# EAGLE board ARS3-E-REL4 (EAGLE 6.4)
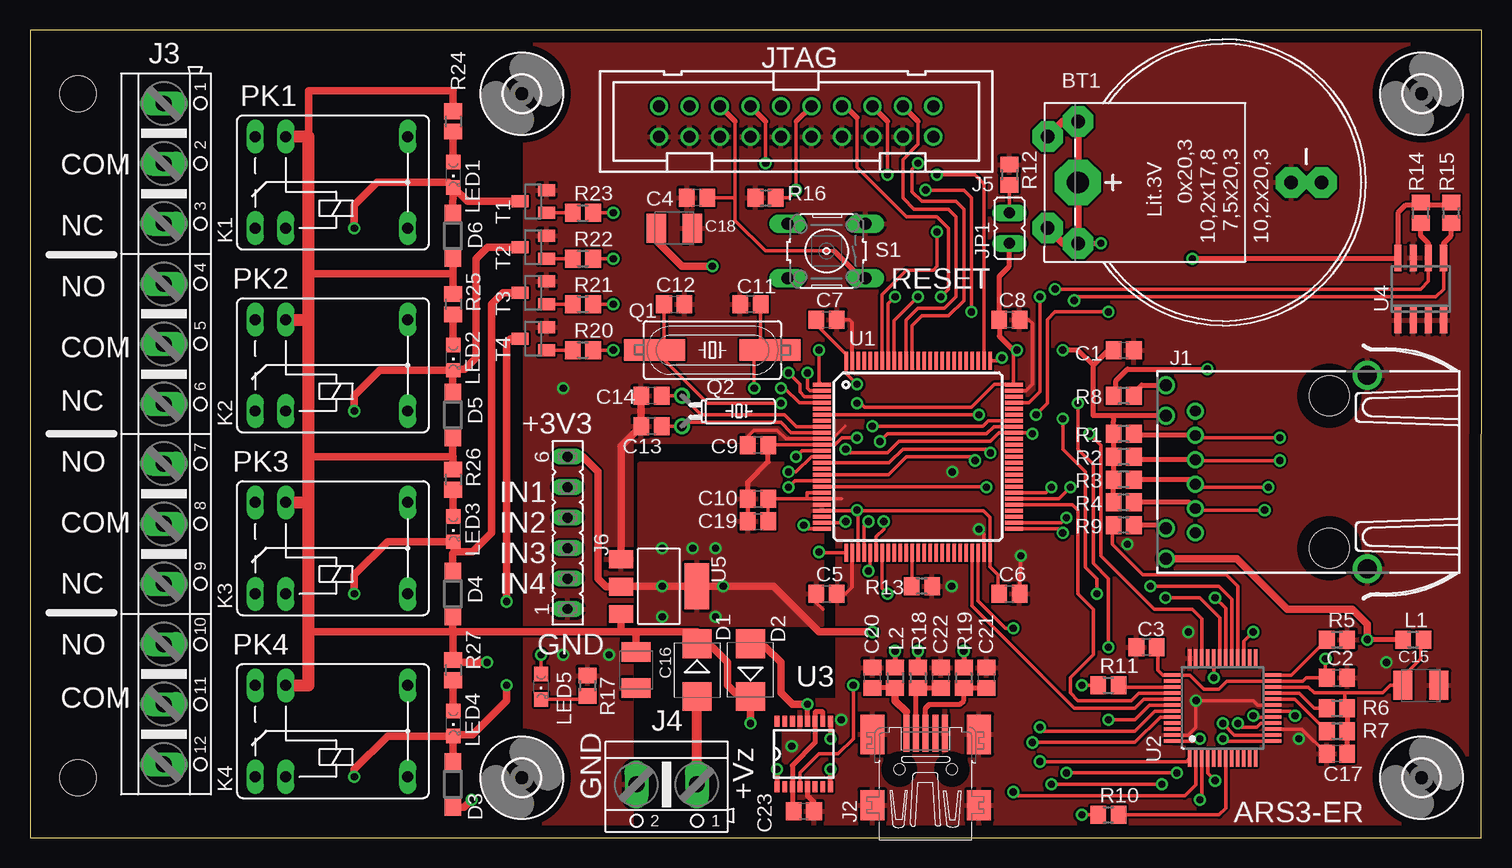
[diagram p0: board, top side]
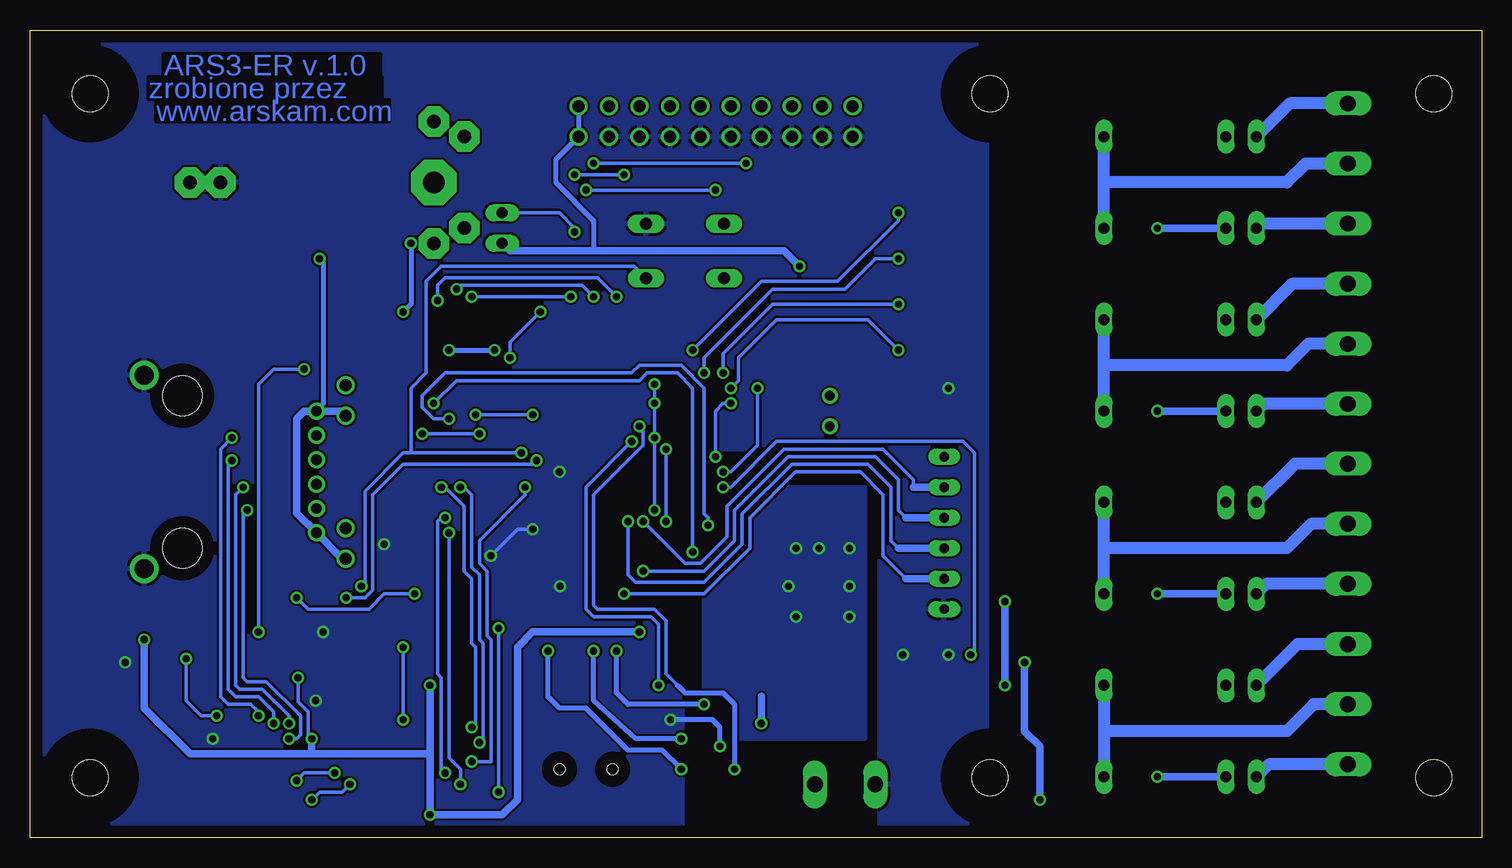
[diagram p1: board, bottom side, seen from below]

Size 121.02 x 67.31 mm. Coordinates in mm from the lower left corner, seen from the top.
Outline: 0,0 121,0 121.02,67.31 0,67.31 0,0
Copper layers (1*16): Top 0.035mm / dielectric 1.5mm / Bottom 0.035mm
Design rules "default *": minimum track width 10mil, minimum drill 19mil, track to track 7mil, track to pad 7mil, pad to pad 7mil, via to via 7mil, smd to smd 7mil, copper to edge 40mil, drill to drill 8mil, minimum pad ring 10mil, minimum via ring 8mil, stop-mask expansion 4mil, vias tented up to drill 0mil, thermal gap 10mil
Holes 3 mm at 4,5 4,62

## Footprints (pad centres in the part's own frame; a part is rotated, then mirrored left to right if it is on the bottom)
B2430UNI = drill 1.118 pad 2.54 octagon: + 3.81,14.605; +@1 -3.81,14.605; +@2 -5.08,12.065; +@3 5.08,12.065; - 0,-5.715; -@1 0,-8.255 | drill 1.803 pad 3.81 octagon: +@4 0,12.065
C0805 = smd 1.3 x 1.5: 1 -0.85,0; 2 0.85,0
SMC_B = smd 1.6 x 2.4: + -1.5,0; - 1.5,0
SMB = smd 2.4 x 2.4: A 2.2,0; C -2.2,0
SOD123 = smd 1.4 x 1.4: A 1.9,0; C -1.9,0
JP = drill 0.9 pad 1.3: 1 5.075,11.18; 2 3.045,11.18; 3 1.015,11.18; 4 -1.015,11.18; 5 -3.045,11.18; 6 -5.075,11.18 | drill 1 pad 1.4: 7 7.23,13.62; 8 4.69,13.62; 9 -4.69,13.62; 10 -7.23,13.62 | drill 1.6 pad 2.184: SH1 -8.065,-3.17; SH2 8.065,-3.17 | hole 3.3: 6.35,0; -6.35,0
32005-201 = smd 3.1 x 0.5: 1 3,1.6; 2 3,0.8; 3 3,0; 4 3,-0.8; 5 3,-1.6 | smd 2.5 x 2: M1 -3,-4.45; M2 -3,4.45 | smd 3.3 x 2: M3 2.9,4.45; M4 2.9,-4.45 | hole 0.9: 0,2.2; 0,-2.2
AK500/12 = drill 1.321 long: 1 -27.534,0; 2 -22.53,0; 3 -17.526,0; 4 -12.497,0; 5 -7.493,0; 6 -2.489,0; 7 2.489,0; 8 7.493,0; 9 12.497,0; 10 17.526,0; 11 22.53,0; 12 27.534,0
AK500/2 = drill 1.321 long: 1 -2.515,0; 2 2.515,0
PAK100/2500-20 = drill 1 pad 1.422: 1 -11.43,-1.27; 2 -11.43,1.27; 3 -8.89,-1.27; 4 -8.89,1.27; 5 -6.35,-1.27; 6 -6.35,1.27; 7 -3.81,-1.27; 8 -3.81,1.27; 9 -1.27,-1.27; 10 -1.27,1.27; 11 1.27,-1.27; 12 1.27,1.27; 13 3.81,-1.27; 14 3.81,1.27; 15 6.35,-1.27; 16 6.35,1.27; 17 8.89,-1.27; 18 8.89,1.27; 19 11.43,-1.27; 20 11.43,1.27
FE06 = drill 0.813 long: 1 -6.35,0; 2 -3.81,0; 3 -1.27,0; 4 1.27,0; 5 3.81,0; 6 6.35,0
JP1 = drill 0.914 long: 1 0,-1.27; 2 0,1.27
FRS1B = drill 0.914 long: 1 0,3.81; 2 0,-3.81; O -2.54,-3.81; P 10.16,3.81; P@ 10.16,-3.81; S -2.54,3.81
R0805 = smd 1.3 x 1.5: 1 -0.85,0; 2 0.85,0
CHIPLED_0805 = smd 1.2 x 1.2: A 0,-1.05; C 0,1.05
SM49 = smd 5.08 x 1.778: 1 -4.826,0; 2 4.826,0
TC26H = drill 0.813: 1 -1.27,0; 2 1.27,0
B3F-10XX = drill 1.016 long: 1 -3.251,2.261; 2 3.251,2.261; 3 -3.251,-2.261; 4 3.251,-2.261
SOT23 = smd 1 x 1.4: 1 -0.95,-1.1; 2 0.95,-1.1; 3 0,1.1
TQFP100 = smd 1.5 x 0.3: 1 -8,6; 2 -8,5.5; 3 -8,5; 4 -8,4.5; 5 -8,4; 6 -8,3.5; 7 -8,3; 8 -8,2.5; 9 -8,2; 10 -8,1.5; 11 -8,1; 12 -8,0.5; 13 -8,0; 14 -8,-0.5; 15 -8,-1; 16 -8,-1.5; 17 -8,-2; 18 -8,-2.5; 19 -8,-3; 20 -8,-3.5; 21 -8,-4; 22 -8,-4.5; 23 -8,-5; 24 -8,-5.5; 25 -8,-6; 51 8,-6; 52 8,-5.5; 53 8,-5; 54 8,-4.5; 55 8,-4; 56 8,-3.5; 57 8,-3; 58 8,-2.5; 59 8,-2; 60 8,-1.5; 61 8,-1; 62 8,-0.5; 63 8,0; 64 8,0.5; 65 8,1; 66 8,1.5; 67 8,2; 68 8,2.5; 69 8,3; 70 8,3.5; 71 8,4; 72 8,4.5; 73 8,5; 74 8,5.5; 75 8,6 | smd 0.3 x 1.5: 26 -6,-8; 27 -5.5,-8; 28 -5,-8; 29 -4.5,-8; 30 -4,-8; 31 -3.5,-8; 32 -3,-8; 33 -2.5,-8; 34 -2,-8; 35 -1.5,-8; 36 -1,-8; 37 -0.5,-8; 38 0,-8; 39 0.5,-8; 40 1,-8; 41 1.5,-8; 42 2,-8; 43 2.5,-8; 44 3,-8; 45 3.5,-8; 46 4,-8; 47 4.5,-8; 48 5,-8; 49 5.5,-8; 50 6,-8; 76 6,8; 77 5.5,8; 78 5,8; 79 4.5,8; 80 4,8; 81 3.5,8; 82 3,8; 83 2.5,8; 84 2,8; 85 1.5,8; 86 1,8; 87 0.5,8; 88 0,8; 89 -0.5,8; 90 -1,8; 91 -1.5,8; 92 -2,8; 93 -2.5,8; 94 -3,8; 95 -3.5,8; 96 -4,8; 97 -4.5,8; 98 -5,8; 99 -5.5,8; 100 -6,8
LQFP48 = smd 1.5 x 0.3: 1 -4.15,2.75; 2 -4.15,2.25; 3 -4.15,1.75; 4 -4.15,1.25; 5 -4.15,0.75; 6 -4.15,0.25; 7 -4.15,-0.25; 8 -4.15,-0.75; 9 -4.15,-1.25; 10 -4.15,-1.75; 11 -4.15,-2.25; 12 -4.15,-2.75; 25 4.15,-2.75; 26 4.15,-2.25; 27 4.15,-1.75; 28 4.15,-1.25; 29 4.15,-0.75; 30 4.15,-0.25; 31 4.15,0.25; 32 4.15,0.75; 33 4.15,1.25; 34 4.15,1.75; 35 4.15,2.25; 36 4.15,2.75 | smd 0.3 x 1.5: 13 -2.75,-4.15; 14 -2.25,-4.15; 15 -1.75,-4.15; 16 -1.25,-4.15; 17 -0.75,-4.15; 18 -0.25,-4.15; 19 0.25,-4.15; 20 0.75,-4.15; 21 1.25,-4.15; 22 1.75,-4.15; 23 2.25,-4.15; 24 2.75,-4.15; 37 2.75,4.15; 38 2.25,4.15; 39 1.75,4.15; 40 1.25,4.15; 41 0.75,4.15; 42 0.25,4.15; 43 -0.25,4.15; 44 -0.75,4.15; 45 -1.25,4.15; 46 -1.75,4.15; 47 -2.25,4.15; 48 -2.75,4.15
SSOP16 = smd 0.914 x 0.406: 1 -2.718,2.223; 2 -2.718,1.587; 3 -2.718,0.953; 4 -2.718,0.318; 5 -2.718,-0.318; 6 -2.718,-0.953; 7 -2.718,-1.587; 8 -2.718,-2.223; 9 2.718,-2.223; 10 2.718,-1.587; 11 2.718,-0.953; 12 2.718,-0.318; 13 2.718,0.318; 14 2.718,0.953; 15 2.718,1.587; 16 2.718,2.223
SO-08 = smd 0.6 x 2.2: 1 -1.905,-2.6; 2 -0.635,-2.6; 3 0.635,-2.6; 4 1.905,-2.6; 5 1.905,2.6; 6 0.635,2.6; 7 -0.635,2.6; 8 -1.905,2.6
SOT223 = smd 1.499 x 2.007: 1 -2.261,-3.15; 2 0.025,-3.15; 3 2.311,-3.15 | smd 3.81 x 2.007: 4 0,3.15
3,0 = hole 3: 0,0

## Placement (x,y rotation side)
BT1  [B2430UNI]  99.42,54.61 90 top
C1  100n  [C0805]  91.17,40.64 0 top
C2  100n  [C0805]  108.95,13.34 0 top
C3  100n  [C0805]  93.08,15.88 180 top
C4  100n  [C0805]  55.61,53.34 180 top
C5  100n  [C0805]  66.41,20.32 0 top
C6  100n  [C0805]  81.64,20.32 0 top
C7  100n  [C0805]  66.41,43.18 0 top
C8  100n  [C0805]  81.64,43.18 0 top
C9  100n  [C0805]  60.69,32.7 180 top
C10  100n  [C0805]  60.69,28.26 0 top
C11  15p  [C0805]  60.05,44.45 180 top
C12  15p  [C0805]  53.7,44.45 0 top
C13  15p  [C0805]  51.8,34.29 180 top
C14  15p  [C0805]  51.8,36.83 180 top
C15  10u/16  [SMC_B]  115.94,12.7 0 top
C16  10u/16  [SMC_B]  50.53,13.97 270 top
C17  100n  [C0805]  108.95,6.99 180 top
C18  10u/16  [SMC_B]  53.7,50.8 0 top
C19  100n  [C0805]  60.69,26.35 0 top
C20  10n  [C0805]  70.22,13.34 90 top
C21  47p  [C0805]  79.74,13.34 90 top
C22  47p  [C0805]  75.93,13.34 90 top
C23  100n  [C0805]  64.5,2.22 0 top
D1  [SMB]  55.61,13.97 270 top
D2  [SMB]  60.05,13.97 90 top
D3  MBR0530T1G  [SOD123]  35.24,4.45 90 top
D4  MBR0530T1G  [SOD123]  35.24,20.32 90 top
D5  MBR0530T1G  [SOD123]  35.24,35.24 90 top
D6  MBR0530T1G  [SOD123]  35.24,50.16 90 top
J1  [JP]  108.31,30.48 90 top
J2  MINI-USB  [32005-201]  74.66,5.71 90 top
J3  [AK500/12]  11.16,33.66 270 top
J4  DG301-5.0/2  [AK500/2]  53.07,4.45 180 top
J5  [PAK100/2500-20]  63.87,59.69 180 top
J6  [FE06]  44.81,25.4 90 top
JP1  ZWORA  [JP1]  81.64,50.8 0 top
K1  HFD41-5  [FRS1B]  21.32,54.61 0 top
K2  HFD41-5  [FRS1B]  21.32,39.37 0 top
K3  HFD41-5  [FRS1B]  21.32,24.13 0 top
K4  HFD41-5  [FRS1B]  21.32,8.89 0 top
L1  1uH  [R0805]  115.3,16.51 0 top
L2  1uH  [R0805]  72.12,13.34 270 top
LED1  [CHIPLED_0805]  35.29,55.24 180 top
LED2  [CHIPLED_0805]  35.29,40.01 180 top
LED3  [CHIPLED_0805]  35.29,25.72 180 top
LED4  [CHIPLED_0805]  35.29,9.53 180 top
LED5  [CHIPLED_0805]  42.6,12.58 180 top
Q1  25MHz  [SM49]  56.88,40.64 0 top
Q2  32,768kHz  [TC26H]  54.34,35.56 270 top
R1  49,9  [R0805]  91.17,33.66 180 top
R2  49,9  [R0805]  91.17,31.75 180 top
R3  49,9  [R0805]  91.17,29.84 180 top
R4  49,9  [R0805]  91.17,27.94 180 top
R5  4k87  [R0805]  108.95,16.51 0 top
R6  2k2  [R0805]  108.95,10.79 0 top
R7  2k2  [R0805]  108.95,8.89 0 top
R8  220  [R0805]  91.17,36.83 180 top
R9  220  [R0805]  91.17,26.04 180 top
R10  2k2  [R0805]  89.9,1.91 0 top
R11  2k2  [R0805]  89.9,12.7 0 top
R12  100k  [R0805]  81.64,55.24 270 top
R13  100k  [R0805]  74.34,20.95 180 top
R14  3k  [R0805]  115.94,52.07 90 top
R15  3k  [R0805]  118.47,52.07 90 top
R16  10k  [R0805]  61.33,53.34 0 top
R17  1k  [R0805]  46.47,12.66 270 top
R18  27  [R0805]  74.03,13.34 270 top
R19  27  [R0805]  77.83,13.34 270 top
R20  3k  [R0805]  46.09,40.64 0 top
R21  3k  [R0805]  46.09,44.45 0 top
R22  3k  [R0805]  46.09,48.26 0 top
R23  3k  [R0805]  46.09,52.07 0 top
R24  1k  [R0805]  35.29,59.69 270 top
R25  1k  [R0805]  35.29,44.45 270 top
R26  1k  [R0805]  35.29,29.84 270 top
R27  1k  [R0805]  35.29,13.97 270 top
S1  [B3F-10XX]  66.41,48.9 180 top
T1  BC847  [SOT23]  41.96,53.02 90 top
T2  BC847  [SOT23]  41.96,49.21 90 top
T3  BC847  [SOT23]  41.96,45.4 90 top
T4  BC847  [SOT23]  41.96,41.59 90 top
U1  STM32F107VC  [TQFP100]  74.03,31.75 0 top
U2  DP83848  [LQFP48]  99.42,10.79 90 top
U3  FT230XS  [SSOP16]  64.5,6.99 90 top
U4  24LC256SN  [SO-08]  115.94,45.72 0 top
U5  LM1117 3V3  [SOT223]  52.44,20.95 270 top
U$5  [3,0]  41,5 0 top
U$6  [3,0]  41,62 0 top
U$7  [3,0]  116,5 0 top
U$8  [3,0]  116,62 0 top

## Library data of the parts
BT1 = battery
C1-C23 L1 L2 R1-R27 = resistor
D1-D6 = diode
J1 = con-pulse; OC_FARNELL: unknown; OC_NEWARK: unknown
J2 = con-cypressindustries; OC_FARNELL: unknown; OC_NEWARK: unknown
J3 J4 = con-ptr500; OC_FARNELL: unknown; OC_NEWARK: unknown
J5 = con-3m; OC_FARNELL: unknown; OC_NEWARK: unknown
J6 = con-lsta; OC_FARNELL: unknown; OC_NEWARK: unknown
JP1 = jumper
K1-K4 = relay; OC_FARNELL: unknown; OC_NEWARK: unknown
LED1-LED5 = led
Q1 Q2 = crystal; OC_FARNELL: unknown; OC_NEWARK: unknown
S1 = switch-omron; MPN: B3F-1000; OC_FARNELL: 176432; OC_NEWARK: 36M3542
T1-T4 = transistor
U1 = stm32-1
U2 = national-semiconductor; MPN: DP83848VYB; OC_FARNELL: 1286817; OC_NEWARK: 11N4484
U3 = ftdichip
U4 = microchip; MF: MICROCHIP; MPN: 24LC256-I/SN; OC_FARNELL: 9757996; OC_NEWARK: 27C9144
U5 = burr-brown; MPN: REG1117 llll; OC_FARNELL: 1097566; OC_NEWARK: 14P6981
U$5-U$8 = holes

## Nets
+5V: C2.1 C3.1 U2.18 U2.23 U2.37
BOOT0: JP1.2 R12.2 U1.94
DP_X1: U1.24 U1.67 U2.34
GND: BT1.- C1.2 C2.2 C3.2 C4.2 C5.2 C6.2 C7.2 C8.2 C9.2 C10.2 C11.2 C12.2 C13.2 C14.2 C15.- C16.- C17.2 C18.- C19.2 C20.2 C21.2 C22.2 C23.2 J1.SH1 J1.SH2 J2.5 J2.M1 J2.M2 J2.M3 J2.M4 J4.2 J5.4 J5.6 J5.8 J5.10 J5.12 J5.14 J5.16 J5.18 J5.20 J6.1 R5.2 R12.1 R13.1 R16.1 R17.1 S1.3 T1.2 T2.2 T3.2 T4.2 U1.10 U1.19 U1.20 U1.27 U1.49 U1.74 U1.99 U2.15 U2.19 U2.35 U2.36 U2.47 U3.5 U3.13 U4.1 U4.2 U4.3 U4.4 U4.7 U5.1
N$1: R10.2 U2.7
N$2: BT1.+ U1.6
N$3: R11.2 U2.39
N$4: J3.3 K1.O
N$5: R5.1 U2.24
N$6: R6.1 U2.21
N$7: J1.2 R1.1 U2.17
N$8: J1.3 R2.1 U2.16
N$9: J1.4 R3.1 U2.14
N$10: J1.5 R4.1 U2.13
N$11: R7.1 U2.20
N$12: J1.7 R8.1
N$13: J1.9 R9.1
N$14: D1.A J4.1
N$15: R8.2 U2.27
N$16: R9.2 U2.28
N$17: C11.1 Q1.2 U1.13
N$18: C12.1 Q1.1 U1.12
N$19: C14.1 Q2.1 U1.8
N$20: C13.1 Q2.2 U1.9
N$21: C23.1 U3.3 U3.10 U3.11
N$22: D2.A L2.1 U3.12
N$23: C20.1 J2.1 L2.2
N$24: C22.1 J2.2 R18.2
N$25: R18.1 U3.9
N$26: C21.1 J2.3 R19.2
N$27: R19.1 U3.8
N$28: J3.2 K1.P K1.P@
N$29: J3.1 K1.S
N$30: D6.A K1.2 LED1.C T1.3
N$31: R23.1 T1.1
N$32: J3.12 K4.O
N$33: J3.11 K4.P K4.P@
N$34: J3.10 K4.S
N$35: D5.A K2.2 LED2.C T2.3
N$36: R22.1 T2.1
N$37: J3.9 K3.O
N$38: J3.8 K3.P K3.P@
N$39: J3.7 K3.S
N$40: D4.A K3.2 LED3.C T3.3
N$41: R21.1 T3.1
N$42: D3.A K4.2 LED4.C T4.3
N$43: R20.1 T4.1
N$44: J3.6 K2.O
N$45: J3.5 K2.P K2.P@
N$46: J3.4 K2.S
N$47: LED1.A R24.2
N$48: LED2.A R25.2
N$49: LED3.A R26.2
N$50: LED4.A R27.2
N$51: LED5.C R17.2
NRST: C4.1 J5.15 S1.1 U1.14 U2.29
PA2: U1.25 U2.30
PA3: U1.26 U2.42
PA4: J6.5 U1.29
PA5: J6.4 U1.30
PA6: J6.3 U1.31
PA7: J6.2 U1.32
PA9: U1.68 U3.4
PA10: U1.69 U3.1
PA13: J5.7 U1.72
PA14: J5.9 R16.2 U1.76
PA15: J5.5 U1.77
PB2: R13.2 U1.37
PB3: J5.13 U1.89
PB4: J5.3 U1.90
PB6: R14.1 U1.92 U4.6
PB7: R15.1 U1.93 U4.5
PB10: U1.47 U2.41
PB11: U1.48 U2.2
PB12: U1.51 U2.3
PB13: U1.52 U2.4
PC1: U1.16 U2.31
PC2: LED5.A U1.17
PC3: U1.18 U2.1
PD8: U1.55 U2.40
PD9: U1.56 U2.43
PD10: U1.57 U2.44
PE2: R23.2 U1.1
PE3: R22.2 U1.2
PE4: R21.2 U1.3
PE5: R20.2 U1.4
V+: C16.+ D1.C D2.C D3.C D4.C D5.C D6.C K1.1 K2.1 K3.1 K4.1 R24.1 R25.1 R26.1 R27.1 U5.3
VCC: C15.+ C17.1 L1.2 R6.2 R7.2 U2.22
ZAS: C1.1 C5.1 C6.1 C7.1 C8.1 C9.1 C10.1 C18.+ C19.1 J1.1 J1.6 J1.8 J1.10 J5.1 J5.2 J6.6 JP1.1 L1.1 R1.2 R2.2 R3.2 R4.2 R10.1 R11.1 R14.2 R15.2 U1.11 U1.21 U1.22 U1.28 U1.50 U1.75 U1.100 U2.32 U2.48 U4.8 U5.2 U5.4

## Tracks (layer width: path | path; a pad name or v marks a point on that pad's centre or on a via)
+5V  (via drill 0.6)
  Top 0.305: U2.18 105.07,10.54 v105.46,10.16 | v108,14.92 108,13.44 C2.1 106.41,13.34 106.12,13.04 U2.23 99.77,13.04 99.11,12.38 97.84,12.38 96.67,13.54 U2.37 94.45,13.54 94.03,13.97 94.03,15.77 C3.1
  Bottom 0.305: v105.46,10.16 106.73,10.16 108,11.43 v108,14.92
BOOT0  (via drill 0.6)
  Top 0.305: U1.94 71.03,45.26 73.07,47.31 75.3,47.31 75.61,47.62 v75.61,50.48 | JP1.2 R12.2
  Bottom 0.305: v75.61,50.48 75.61,50.8 76.88,52.07 JP1.2
DP_X1  (via drill 0.6)
  Top 0.305: v67.99,32.38 67.99,32.07 71.48,32.07 72.44,33.02 80.06,33.02 80.79,33.75 U1.67 83.45,33.75 v83.55,33.66 | v67.99,26.35 67.89,26.25 U1.24 | U2.34 97.67,18.26 96.89,19.05 93.71,19.05 89.27,23.5 89.27,32.7 v88.31,33.66
  Bottom 0.305: v67.99,32.38 v67.99,26.35 | v83.55,33.66 v88.31,33.66
GND  (via drill 0.6)
  Top 0.254: U1.10 66.91,33.25 67.94,34.29
  Top 0.305: U2.15 106.04,9.04 C17.2 108.31,6.99 | U2.19 102.35,11.04 101.97,11.43 v97.2,11.43 97.2,9.21 96.54,8.54 U2.47 | U1.10 63,33.25 62.28,33.97 60.37,33.97 59.74,33.34 59.74,32.8 C9.2 | U1.74 83.02,37.25 83.55,37.78 83.55,42.86 83.23,43.18 C8.2 | U1.99 68.53,42.97 68.31,43.18 C7.2 | U1.27 68.53,20.85 67.99,20.32 C5.2 | U1.49 79.53,25.3 v79.11,25.72 | v82.6,23.5 C6.2 | 64.77,28.26 66.02,28.26 U1.20 67.63,28.26 | 64.77,28.26 C10.2 C19.2 | U1.19 64.77,28.75 64.77,28.26
  Top 0.406: U3.5 64.82,3.49 65.35,2.96 C23.2
  Top 0.61: C14.2 C13.2 49.28,32.62 U5.1
  Bottom 0.305: v79.11,25.72 80.38,25.72 v82.6,23.5
  Bottom 0.406: v63.5,7.62 63.5,9.21 64.14,9.84 v67.63,9.84
  other vias: 113.08,14.61 96.57,17.14 105.78,8.26 91.49,24.45 76.83,20.95 44.45,37.47 76.88,30.48 44.45,15.24 48.26,15.24
  pour Bottom: 121.28,67.31 41.27,67.31 41.27,0 50.16,0 50.16,32.38 66.67,32.38 120.65,0 120.65,15.88 121.28,15.88
  pour Top: 120.65,67.31 41.27,67.31 41.27,66.67 41.27,0 50.16,0 50.16,33.02 67.31,33.02 67.31,32.38 67.31,11.43 63.5,11.43 62.87,11.43 62.87,0 121.28,0 121.28,67.31
  pour Bottom: 120.65,67.31 41.27,67.31 41.27,66.67 41.27,0 50.16,0 50.16,33.02 66.04,33.02 66.67,33.02 66.67,0 121.28,0 121.28,67.31
N$1
  Top 0.305: U2.7 99.67,2.47 99.11,1.91 R10.2
N$2  (via drill 0.6)
  Top 0.305: U1.6 79.1,35.25 v79.11,35.24 | v83.87,35.24 84.82,36.2 84.82,43.18 85.45,43.81 v89.9,43.81
  Top 0.406: 87.36,49.53 v89.27,49.53
  Top 0.61: BT1.+ 86.09,59.69 87.36,59.69 87.36,49.53 86.09,49.53 84.82,50.8
  Bottom 0.305: v79.11,35.24 v83.87,35.24
  Bottom 0.406: v89.27,49.53 89.27,44.45 v89.9,43.81
N$3
  Top 0.305: U2.39 90.91,12.54 R11.2
N$4
  Bottom 1.016: J3.3 18.4,51.18 K1.O
N$5
  Top 0.305: U2.24 105.14,13.54 R5.1
N$6
  Top 0.305: U2.21 105.8,12.04 107.05,10.79 R6.1
N$7  (via drill 0.6)
  Top 0.305: U2.17 102.08,10.04 v101.97,10.16 | v104.19,33.34 97.32,33.34 J1.2
  Top 0.406: J1.2 92.15,33.52 R1.1
  Bottom 0.305: v101.97,10.16 101.97,10.48 102.6,11.11 104.5,11.11 105.14,11.75 105.14,32.38 v104.19,33.34
N$8  (via drill 0.6)
  Top 0.305: U2.16 102.62,9.54 102.28,9.21 101.01,9.21 v100.69,9.53 | v104.19,31.43 97.2,31.43 J1.3
  Top 0.406: J1.3 92.28,31.5 R2.1
  Bottom 0.305: v100.69,9.53 100.69,10.48 101.97,11.75 103.87,11.75 104.5,12.38 104.5,31.11 v104.19,31.43
N$9  (via drill 0.6)
  Top 0.305: U2.14 100.41,8.54 v99.42,9.53 | v103.23,29.21 97.52,29.21 J1.4
  Top 0.406: J1.4 96.75,29.84 R3.1
  Bottom 0.305: v99.42,9.53 99.42,10.16 101.65,12.38 103.55,12.38 103.87,12.7 103.87,28.57 v103.23,29.21
N$10  (via drill 0.6)
  Top 0.305: U2.13 99.64,8.04 v99.42,8.26 | v102.92,27.3 97.27,27.3 J1.5
  Top 0.406: J1.5 96.63,27.94 R4.1
  Bottom 0.305: v99.42,8.26 98.79,8.26 98.47,8.57 98.47,10.16 101.33,13.02 102.92,13.02 103.23,13.34 103.23,26.99 v102.92,27.3
N$11
  Top 0.305: U2.20 105.44,11.54 R7.1
N$12
  Top 0.406: R8.1 92.44,37.25 92.44,37.47 92.69,37.71 J1.7
N$13
  Top 0.406: J1.9 94.45,26.04 R9.1
N$14
  Top 0.61: 55.59,11.77 D1.A
  Top 0.813: J4.1 55.59,11.77
N$15  (via drill 0.6)
  Top 0.305: U2.27 101.17,16.36 v101.97,17.14
  Top 0.406: R8.2 90.53,37.05 90.53,38.1 91.49,39.05 v98.16,39.05
  Bottom 0.305: v101.97,17.14 101.97,37.78 100.69,39.05 v98.16,39.05
N$16
  Top 0.305: U2.28 100.67,20.98 99.74,21.91 92.76,21.91 90.22,24.45 90.22,25.93 R9.2
N$17  (via drill 0.6)
  Top 0.305: U1.13 65.14,31.75 63.87,30.48 v63.23,30.48 | C11.1 60.91,41.44 Q1.2 61.96,40.39 61.26,40.39 61.01,40.64 60.37,40.01 v60.37,37.47
  Bottom 0.305: v63.23,30.48 62.59,30.48 60.37,32.7 v60.37,37.47
N$18  (via drill 0.6)
  Top 0.305: U1.12 64.36,32.25 v63.87,31.75 | v62.59,36.2 56.5,36.2 Q1.1 52.44,40.64 52.85,41.06 C12.1
  Bottom 0.305: v63.87,31.75 63.87,35.56 63.23,36.2 v62.59,36.2
N$19
  Top 0.305: U1.8 63.91,34.25 62.91,35.24 55.93,35.24 Q2.1 C14.1
N$20
  Top 0.305: U1.9 63.45,33.75 62.59,34.61 54.66,34.61 Q2.2 C13.1
N$21
  Top 0.406: U3.10 66.09,10.48 65.45,10.48 U3.11 65.45,7.94 63.55,6.03 U3.3 63.55,2.33 C23.1
N$22  (via drill 0.6)
  Top 0.406: U3.12 v64.82,11.11 | v72.12,15.56 L2.1
  Top 0.61: D2.A 60.35,15.88 61.33,15.88 62.59,14.61 62.59,12.06 63.55,11.11 v64.82,11.11
  Bottom 0.406: v64.82,11.11 71.17,11.11 72.12,12.06 v72.12,15.56
N$23
  Top 0.406: L2.2 C20.1
  Top 0.508: J2.1 73.06,10.49
  Top 0.61: 73.06,10.49 72.12,11.43 L2.2
N$24
  Top 0.406: J2.2 73.86,12.32 R18.2 C22.1
N$25  (via drill 0.6)
  Top 0.406: U3.9 v66.72,8.26 | v74.03,15.56 R18.1
  Bottom 0.406: v66.72,8.26 70.53,8.26 74.03,11.43 v74.03,15.56
N$26
  Top 0.406: J2.3 74.66,10.79 74.98,11.11 77.52,11.11 77.83,11.43 R19.2 C21.1
N$27  (via drill 0.6)
  Top 0.406: U3.8 v66.72,5.71 | v77.83,15.56 R19.1
  Bottom 0.406: v66.72,5.71 68.31,7.3 71.17,7.3 74.66,10.79 76.88,10.79 77.83,11.75 v77.83,15.56
N$28
  Bottom 1.016: K1.P@ 31.48,54.61 | 31.48,54.61 K1.P | J3.2 14.66,56.19 16.24,54.61 31.48,54.61
N$29
  Bottom 1.016: J3.1 16.01,61.19 K1.S
N$30  (via drill 0.6)
  Top 0.61: T1.3 36.46,53.02 LED1.C | LED1.C 34.88,54.61 28.94,54.61 27.04,52.7 v27.04,50.8 | 35.24,54.15 LED1.C | D6.A LED1.C
  Bottom 0.61: v27.04,50.8 K1.2
N$31
  Top 0.305: R23.1 T1.1
N$32
  Bottom 1.016: J3.12 17.74,6.12 K4.O
N$33
  Bottom 1.016: K4.P 31.48,8.89 | 31.48,8.89 K4.P@ | J3.11 14.01,11.12 16.24,8.89 31.48,8.89
N$34
  Bottom 1.016: J3.10 15.35,16.13 K4.S
N$35  (via drill 0.6)
  Top 0.61: T2.3 38.15,49.21 37.2,48.26 37.2,40.01 36.24,39.05 35.39,39.05 LED2.C | LED2.C 29.16,38.95 27.04,36.83 v27.04,35.56 | LED2.C 35.24,38.91 D5.A
  Bottom 0.61: v27.04,35.56 K2.2
N$36
  Top 0.305: R22.1 T2.1
N$37
  Bottom 1.016: J3.9 17.94,21.16 K3.O
N$38
  Bottom 1.016: K3.P@ 31.48,24.13 | 31.48,24.13 K3.P | J3.8 14.21,26.16 16.24,24.13 31.48,24.13
N$39
  Bottom 1.016: J3.7 15.55,31.17 K3.S
N$40  (via drill 0.6)
  Top 0.61: T3.3 39.42,45.4 38.47,44.45 38.47,25.4 36.88,23.81 35.39,23.81 | 35.39,23.81 LED3.C 29.8,24.67 27.04,21.91 v27.04,20.32 | D4.A 35.24,23.67 35.39,23.81
  Bottom 0.61: v27.04,20.32 K3.2
N$41
  Top 0.305: R21.1 T3.1
N$42  (via drill 0.6)
  Top 0.61: T4.3 40.05,41.59 39.73,41.27 v39.73,19.68 | LED4.C 29.8,8.47 27.04,5.71 v27.04,5.08 | v39.73,12.7 39.73,11.43 36.88,8.57 35.39,8.57 LED4.C | D3.A 35.29,6.34 LED4.C
  Bottom 0.61: v27.04,5.08 K4.2 | v39.73,19.68 v39.73,12.7
N$43
  Top 0.305: R20.1 T4.1
N$44
  Bottom 1.016: J3.6 18.2,36.14 K2.O
N$45
  Bottom 1.016: J3.5 14.46,41.15 16.24,39.37 31.48,39.37 | 31.48,39.37 K2.P | K2.P@ 31.48,39.37
N$46
  Bottom 1.016: J3.4 15.81,46.15 K2.S
N$47
  Top 0.61: R24.2 LED1.A
N$48
  Top 0.61: R25.2 LED2.A
N$49
  Top 0.61: R26.2 LED3.A
N$50
  Top 0.61: R27.2 LED4.A
N$51
  Top 0.305: LED5.C 46.19,11.53 R17.2
NRST  (via drill 0.6)
  Top 0.305: U1.14 71.62,31.25 72.75,32.38 79.74,32.38 v80.06,32.07 | v93.39,20.95 99.11,20.95 100.17,19.89 U2.29 | 58.78,59.69 58.78,53.34 | 58.78,53.34 58.78,51.44 61.33,48.9 67.04,48.9 | 69.3,46.63 S1.1 | C4.1 58.78,53.34
  Top 0.406: J5.15 58.78,59.69 | 67.04,48.9 69.3,46.63
  Bottom 0.305: v80.06,32.07 89.27,32.07 | 89.27,32.07 89.9,32.07 93.08,28.89 93.08,21.27 v93.39,20.95 | S1.1 70.65,47.62 86.72,47.62 88,46.35 88,38.73 89.27,37.47 89.27,32.07
PA2  (via drill 0.6)
  Top 0.305: U1.25 64.78,25.75 v64.5,26.04 | v86.09,34.92 86.09,32.38 88,30.48 88,22.54 88.95,21.59 v88.95,20.32 | v98.79,20 99.67,19.12 U2.30
  Bottom 0.305: v64.5,26.04 64.5,26.67 64.82,26.99 64.82,37.47 66.72,39.37 70.22,39.37 70.85,38.73 86.41,38.73 88.31,36.83 88.31,35.88 87.36,34.92 v86.09,34.92 | v88.95,20.32 91.49,20.32 92.76,19.05 97.84,19.05 v98.79,20
PA3  (via drill 0.6)
  Top 0.305: U1.26 65.77,23.75 v65.77,23.81 | v87.36,36.2 87.36,32.38 88.63,31.11 88.63,22.86 89.9,21.59 v89.9,15.88 | v89.9,9.84 92.12,9.84 93.33,11.04 U2.42
  Bottom 0.305: v65.77,23.81 65.77,37.47 67.04,38.73 69.58,38.73 70.22,38.1 85.45,38.1 v87.36,36.2 | v89.9,15.88 v89.9,9.84
PA4  (via drill 0.6)
  Top 0.305: U1.29 69.53,25.98 v69.9,26.35
  Bottom 0.305: v69.9,26.35 66.41,22.86 65.14,22.86 62.91,25.08 62.91,27.62 58.15,32.38 49.9,32.38 47.35,29.84 47.35,29.21
  Bottom 0.61: 47.35,29.21 J6.5
PA5  (via drill 0.6)
  Top 0.305: U1.30 70.03,22.35 v69.9,22.23
  Bottom 0.305: v69.9,22.23 64.82,22.23 62.28,24.77 62.28,27.3 57.83,31.75 50.53,31.75 48.62,29.84 48.62,27.3 47.99,26.67
  Bottom 0.61: 47.99,26.67 J6.4
PA6  (via drill 0.6)
  Top 0.305: U1.31 70.53,25.07 71.17,25.72 v71.17,26.35
  Bottom 0.305: v71.17,26.35 71.17,21.91 70.53,21.27 64.82,21.27 61.64,24.45 61.64,26.99 57.52,31.11 51.16,31.11 49.26,29.21 49.26,24.77 48.62,24.13
  Bottom 0.61: 48.62,24.13 J6.3
PA7  (via drill 0.6)
  Top 0.305: U1.32 71.03,20.78 v71.48,20.32
  Bottom 0.305: v71.48,20.32 64.82,20.32 61.01,24.13 61.01,26.67 57.2,30.48 51.8,30.48 49.9,28.57 49.9,23.5 47.99,21.59
  Bottom 0.61: J6.2 47.99,21.59
PA9  (via drill 0.6)
  Top 0.305: v70.85,33.02 71.48,33.66 79.74,33.66 80.33,34.25 U1.68 | v68.63,12.7 68.63,8.26 67.36,6.99 65.77,6.99 64.18,5.4 U3.4
  Bottom 0.305: v70.85,33.02 74.66,29.21 74.66,19.05 74.03,18.41 69.26,18.41 68.63,17.78 v68.63,12.7
PA10  (via drill 0.6)
  Top 0.305: v70.22,34.29 79.42,34.29 79.88,34.75 U1.69
  Top 0.406: v62.28,5.71 U3.1
  Bottom 0.305: v70.22,34.29 69.9,33.97 69.9,32.7 74.03,28.57 74.03,19.37 73.71,19.05 68.94,19.05 67.99,18.1 67.99,13.65 67.04,12.7
  Bottom 0.406: 67.04,12.7 66.41,12.06 63.23,12.06 62.28,11.11 v62.28,5.71
PA13  (via drill 0.6)
  Top 0.305: v84.19,45.09 84.19,37.15 83.29,36.25 U1.72 | 68.94,60.01 68.94,55.88 73.07,51.75 75.61,51.75 76.56,50.8 76.56,45.72 v75.93,45.09 | 67.99,60.96 J5.7
  Top 0.406: 68.94,60.01 67.99,60.96
  Bottom 0.305: v84.19,45.09 v75.93,45.09
PA14  (via drill 0.6)
  Top 0.305: U1.76 80.75,39.75 v81.01,40.01 | v78.47,43.81 78.47,53.34 77.83,53.98 v74.66,53.98 | 63.87,59.69 v63.87,53.98 63.23,53.34 R16.2
  Top 0.406: 63.87,59.69 J5.9
  Bottom 0.305: v81.01,40.01 81.01,41.27 v78.47,43.81 | v74.66,53.98 v63.87,53.98
PA15  (via drill 0.6)
  Top 0.305: U1.77 79.53,54.51 78.79,55.24 v75.61,55.24 | v71.48,55.24 71.48,59.69
  Top 0.406: 71.48,59.69 J5.5
  Bottom 0.305: v75.61,55.24 v71.48,55.24
PB2
  Top 0.305: U1.37 73.53,20.99 R13.2
PB3  (via drill 0.6)
  Top 0.305: v74.03,56.2 73.53,55.7 73.53,53.84 74.34,53.02 77.2,53.02 77.83,52.39 77.83,44.77 76.56,43.5 74.34,43.5 73.53,42.68 U1.89 | v61.33,56.2 61.33,59.69
  Top 0.406: 61.33,59.69 J5.13
  Bottom 0.305: v74.03,56.2 v61.33,56.2
PB4
  Top 0.305: U1.90 73.03,43.13 74.03,44.13 76.25,44.13 77.2,45.09 77.2,51.75 76.56,52.39 73.71,52.39 72.75,53.34 72.75,56.52 74.03,57.78 74.03,59.69
  Top 0.406: 74.03,59.69 J5.3
PB6  (via drill 0.6)
  Top 0.305: U1.92 72.03,43.09 v74.03,45.09 | v85.45,45.72 115.94,45.72 116.57,46.35 U4.6
  Top 0.406: U4.6 116.57,49.53 115.94,50.16 R14.1
  Bottom 0.305: v74.03,45.09 74.98,46.04 85.14,46.04 v85.45,45.72
PB7  (via drill 0.6)
  Top 0.305: U1.93 71.53,44.49 v72.12,45.09 | U4.5 117.84,45.72 117.2,45.09 87.36,45.09 v87.04,44.77
  Top 0.406: U4.5 117.84,49.53 118.47,50.16 R15.1
  Bottom 0.305: v72.12,45.09 73.71,46.67 86.41,46.67 87.04,46.04 v87.04,44.77
PB10
  Top 0.305: U2.41 92.87,11.54 92.12,10.79 87.04,10.79 78.53,19.31 U1.47
PB11  (via drill 0.6)
  Top 0.305: U1.48 79.03,19.77 81.33,17.46 v81.96,17.46 | U2.2 97.17,4.42 96.25,3.49 82.28,3.49 v81.96,3.81
  Bottom 0.305: v81.96,17.46 v81.96,3.81
PB12  (via drill 0.6)
  Top 0.305: U1.51 85.74,25.75 v86.09,25.4 | v85.14,4.45 v94.34,4.45 | v97.52,3.17 97.52,3.49 97.67,3.65 U2.3
  Bottom 0.305: v86.09,25.4 86.09,6.67 85.14,5.71 v85.14,4.45 | v94.34,4.45 94.98,3.81 96.89,3.81 v97.52,3.17
PB13  (via drill 0.6)
  Top 0.305: U1.52 85.99,26.25 v86.41,26.67 | v86.41,5.4 v95.61,5.4 | U2.4 98.17,5.38 v98.79,4.76
  Bottom 0.305: v86.41,26.67 86.72,26.67 87.04,26.35 87.04,13.65 86.72,13.34 86.72,5.71 v86.41,5.4 | v95.61,5.4 98.16,5.4 v98.79,4.76
PC1  (via drill 0.6)
  Top 0.305: v78.79,31.43 78.47,31.75 73.07,31.75 71.57,30.25 U1.16 | v94.66,20 97.52,20 99.17,18.35 U2.31
  Bottom 0.305: v78.79,31.43 79.11,31.11 89.9,31.11 92.44,28.57 92.44,20.64 93.08,20 v94.66,20
PC2  (via drill 0.6)
  Top 0.305: U1.17 63.77,29.75 v63.23,29.21 | v42.59,15.24 LED5.A
  Bottom 0.305: v63.23,29.21 62.59,29.21 58.78,33.02 43.23,33.02 42.27,32.07 42.27,15.56 v42.59,15.24
PC3  (via drill 0.6)
  Top 0.305: U1.18 79.74,29.25 v79.74,29.21 | v84.19,6.35 96.38,6.35 U2.1
  Bottom 0.305: v79.74,29.21 79.74,28.57 83.55,24.77 83.55,22.86 82.92,22.23 82.92,16.83 82.6,16.51 82.6,6.35 v84.19,6.35
PD8
  Top 0.305: U2.40 92.42,12.04 91.81,11.43 87.36,11.43 86.72,12.06 86.72,13.34 88.63,15.24 88.63,19.05 87.36,20.32 87.36,27.3 86.92,27.75 U1.55
PD9  (via drill 0.6)
  Top 0.305: U1.56 85.77,28.25 v86.72,29.21 | U2.43 93.78,10.54 92.12,8.89 84.5,8.89 v84.19,9.21
  Bottom 0.305: v86.72,29.21 86.41,29.21 84.82,27.62 84.82,22.23 84.19,21.59 84.19,16.19 83.87,15.88 83.87,9.53 v84.19,9.21
PD10  (via drill 0.6)
  Top 0.305: U1.57 84.68,28.75 v85.14,29.21 | v83.55,7.94 92.12,7.94 94.23,10.04 U2.44
  Bottom 0.305: v85.14,29.21 84.82,29.21 84.19,28.57 84.19,22.54 83.55,21.91 83.55,16.51 83.23,16.19 83.23,8.26 v83.55,7.94
PE2  (via drill 0.6)
  Top 0.305: U1.1 65.77,38.01 v65.77,40.64 | v48.62,52.07 R23.2
  Bottom 0.305: v65.77,40.64 60.05,46.35 53.7,46.35 48.62,51.44 v48.62,52.07
PE3  (via drill 0.6)
  Top 0.305: U1.2 65.03,37.25 64.82,37.47 v64.82,38.73 | v48.62,48.26 R22.2
  Bottom 0.305: v64.82,38.73 64.82,40.01 59.1,45.72 53.07,45.72 50.53,48.26 v48.62,48.26
PE4  (via drill 0.6)
  Top 0.305: U1.3 64.58,36.75 64.18,37.15 64.18,37.78 v63.23,38.73 | v48.62,44.45 R21.2
  Bottom 0.305: v63.23,38.73 63.23,40.32 59.1,44.45 v48.62,44.45
PE5  (via drill 0.6)
  Top 0.305: U1.4 64.13,36.25 62.91,37.47 v62.59,37.47 | v48.62,40.64 R20.2
  Bottom 0.305: v62.59,37.47 61.96,38.1 61.96,40.01 58.78,43.18 51.16,43.18 v48.62,40.64
V+  (via drill 0.6)
  Top 0.61: 49.06,18.41 U5.3 49.26,18.64 49.26,17.14 | v60.05,9.53 D2.C 60.05,12.06 58.78,12.06 58.15,12.7 58.15,14.61 56.88,15.88 55.91,15.88 D1.C 55.61,17.14 50.53,17.14 | 50.53,17.14 49.26,17.14 | C16.+ 50.53,17.14 | R26.1 35.29,31.75 | 35.29,31.75 23.23,31.75 | 49.26,17.14 35.29,17.14 | 35.29,17.14 23.23,17.14 | R25.1 35.29,46.99 | 35.29,46.99 23.23,46.99 | R24.1 35.29,62.23 23.23,62.23 23.23,58.42 | 35.29,17.14 R27.1 35.51,14.61 v38.1,14.61 | D3.C 36.2,2.54 v36.83,3.17 | D4.C 35.24,17.19 35.29,17.14 | D5.C 35.24,31.8 35.29,31.75 | D6.C 35.29,46.99
  Top 1.016: K4.1 23.23,12.7 23.23,17.14 23.23,27.94 | 23.23,27.94 23.23,31.75 23.23,43.18 | 23.23,43.18 23.23,46.99 23.23,58.42 K1.1 | K2.1 23.23,43.18 | K3.1 23.23,27.94
  Bottom 0.61: D2.C v60.05,9.53 | v36.83,3.17 36.83,7.62 38.1,8.89 v38.1,14.61
VCC
  Top 0.305: U2.22 106.56,12.54 107.05,12.06 109.58,12.06 | 109.58,12.06 109.58,11.01 R6.2 | 109.58,12.06 112.76,12.06 113.39,12.7 C15.+ 114.44,13.42 115.94,14.92 115.94,16.3 L1.2
  Top 0.406: R6.2 R7.2 C17.1
ZAS  (via drill 0.6)
  Top 0.305: U2.32 v98.67,13.34 | C9.1 61.59,32.75 U1.11 67.09,32.75 67.67,33.34 v68.94,33.34 | 81.96,40.64 81.96,37.81 81.99,37.78 | C7.1 65.77,42.97 65.77,42.55 68.03,40.29 U1.100 68.03,38.7 v68.94,37.78 | 81.99,37.78 U1.75 | U1.22 68.89,27.25 | 68.89,27.25 79.48,27.25 80.03,26.7 U1.50 80.03,22.57 80.69,21.91 80.69,20.42 C6.1 | 68.89,27.25 v68.94,27.3 69.03,27.23 U1.28 | 66.09,19.05 65.45,19.68 65.45,20.22 C5.1 | R10.1 v87.68,1.91 | R11.1 v87.68,12.7 | 81.99,37.78 80.38,37.78 78.47,35.88 69.58,35.88 69.26,36.2 v68.94,36.2 | C19.1 C10.1 | U2.48 97.31,8.04 v97.52,8.26
  Top 0.406: J1.8 90.29,35.17 | 90.29,35.17 90.32,34.71 R1.2 R2.2 | R2.2 90.53,31.75 | R4.2 R3.2 R2.2 | JP1.1 81.64,47.62 80.8,46.77 C8.1 80.8,41.81 81.96,40.64 v82.28,40.64 | L1.1 v111.49,16.51 | 90.29,35.17 88.63,35.17 88.63,39.37 | 88.63,39.37 89.9,40.64 C1.1 | v96.89,48.26 113.97,48.26 U4.8 114.03,52.07 114.67,52.7 115.94,52.7 | R15.2 118.26,52.7 115.94,52.7 | 88.63,39.37 87.36,40.64 v86.09,40.64 | C10.1 59.84,29.63 61.54,31.33 C9.1 | R14.2 115.94,52.7
  Top 0.61: v111.49,16.51 111.49,17.78 110.22,19.05 104.82,19.05 100.62,23.25 J1.10 | C18.+ 52.44,50.57 52.44,49.53 54.34,47.62 v56.88,47.62 | v70.22,17.14 65.77,17.14 61.96,20.95 U5.4 49.31,20.95 U5.2 48.02,20.93 47.35,21.59 47.35,30.48 46.09,31.75 J6.6
  Bottom 0.305: v97.52,8.26 97.84,8.57 97.84,10.48 98.67,11.31 v98.67,13.34 | v68.94,37.78 v68.94,36.2 v68.94,33.34 v68.94,27.3 68.94,27.25 | 96.89,35.56 J1.1
  Bottom 0.406: J5.1 J5.2 77.2,56.52 77.2,54.61 74.03,51.44 74.03,48.9 | v96.89,48.26 96.57,47.94 96.57,36.2 97.14,35.63 J1.1 | v86.09,40.64 v82.28,40.64
  Bottom 0.61: J1.1 95.08,35.55 J1.8 | v87.68,12.7 87.68,6.99 | 87.68,6.99 v87.68,1.91 81.64,1.91 80.38,3.17 80.38,15.88 79.11,17.14 v70.22,17.14 | 96.89,35.56 98.16,35.56 98.79,34.92 98.79,27.06 J1.6 94.98,23.25 J1.10 | v111.49,16.51 111.49,10.79 107.68,6.99 97.52,6.99 | 97.52,6.99 87.68,6.99 | v97.52,8.26 97.52,6.99 | v56.88,47.62 58.15,48.9 74.03,48.9 81.01,48.9 JP1.1
  other vias: 55.24,24.13 57.15,24.13 57.78,20.95 57.15,18.41 52.7,20.95 52.7,24.13 52.7,18.41
  pour Top: 50.8,29.21 50.8,17.78 66.04,17.78 66.04,31.11 50.8,31.11
  pour Bottom: 51.44,29.21 51.44,8.26 64.77,8.26 64.77,29.21

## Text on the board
Bottom: ARS3-ER v.1.0 | zrobione przez | www.arskam.com
tNames: JTAG | PK1 | COM | NC | PK2 | RESET | NO | COM | NC | +3V3 | NO | PK3 | IN1 | COM | IN2 | IN3 | NC | IN4 | NO | PK4 | GND | COM | GND | +Vz | ARS3-ER | warstwy 51, 52 wylaczone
